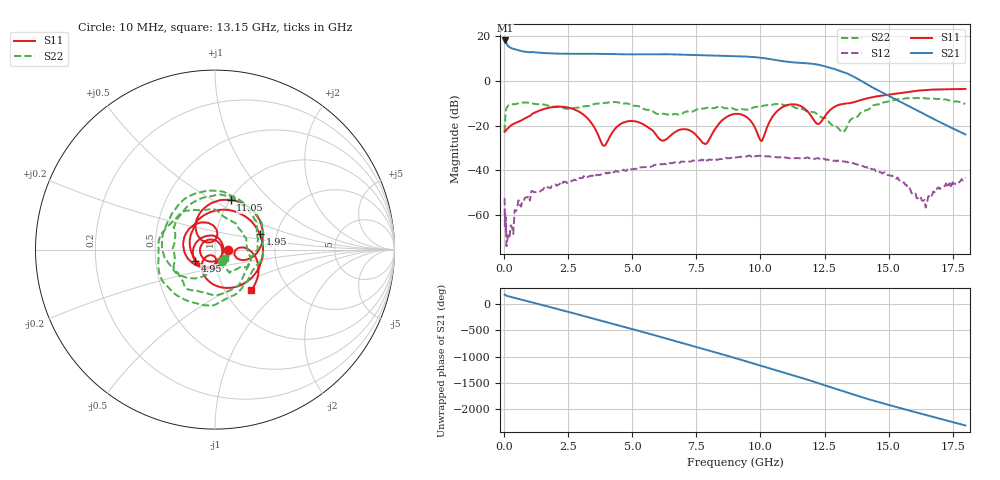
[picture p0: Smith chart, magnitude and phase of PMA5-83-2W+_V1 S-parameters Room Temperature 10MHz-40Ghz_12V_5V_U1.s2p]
!Mini-Circuits Laboratory
!S-Parameters
!Model: US-AMP-1
!Run / Lot / Date Code: N/A /  / N/A
!Fixture: ON TB-
!Network Analyzer: NFA N8975A;  Serial number: 74408
!Date: 12/1/2023 at 8:03:08 AM
!No.: Unit# 1 (#1)
!Tested with:
!Condition 2: Vdd = +12V; Vg2= +5V; Idd= 400mA
# Hz  S  dB  R  50
!Frequency  S11 dB  S11 Deg  S21 dB  S21 Deg  S12 dB  S12 Deg  S22 dB  S22 Deg
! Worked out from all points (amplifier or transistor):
!   368 points, 10 MHz to 18 GHz, reference 50 ohm
!   highest |S21| = 18.2 dB at 20 MHz (marker M1)
!   |S21| within 3 dB of that: start of sweep to 198.7 MHz
!   unconditionally stable (mu >= 1): start of sweep to end of sweep
!   at 2.7 GHz: K = 18.17, MAG = 12.7 dB, |S12| = -44.5 dB
!   at 8.85 GHz: K = 6.53, MAG = 11.6 dB, |S12| = -34.3 dB
!   at 18 GHz: K = 559.16, MAG = -20.9 dB, |S12| = -43.1 dB
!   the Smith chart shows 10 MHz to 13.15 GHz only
!   S11 on the Smith chart (normalised r, x): 10 MHz: 1.16, -0.00; 1.95 GHz: 1.63, +0.30; 4.95 GHz: 0.79, -0.10; 11.05 GHz: 1.01, +0.61; 13.15 GHz: 1.31, -0.66
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1e7  -22.68 -0.5  17.95 177.8  -52.38 -62.5  -22.73 -57.9
2e7  -22.62 -3.8  18.17 174.4  -65.67 23.9  -19.73 -85.4
4.5e8  -18.71 -130.9  14.12 108.2  -58.23 52.9  -10.29 145.9
1.1e9  -14.57 124.1  13.01 27.2  -49.12 -39.4  -10.05 72.8
1.95e9  -11.56 18.7  12.33 -81.3  -46.48 -144.7  -11.47 -1.4
2.55e9  -12.01 -47.0  12.22 -158.0  -45.09 138.9  -12.26 -36.4
3.05e9  -14.69 -98.4  12.22 137.2  -43.40 76.6  -11.40 -60.0
4.05e9  -26.41 -85.3  12.09 5.7  -40.94 -45.2  -9.56 -130.2
4.95e9  -17.86 -151.1  11.95 -112.5  -39.45 -157.2  -10.56 154.9
5.5e9  -19.85 142.9  12.01 174.6  -38.47 130.5  -12.70 106.2
6.05e9  -25.89 33.6  12.04 100.4  -37.19 62.9  -14.71 60.9
6.75e9  -22.21 -127.0  11.91 4.7  -36.63 -29.8  -14.91 14.5
7.4e9  -23.22 130.4  11.65 -84.3  -35.61 -113.8  -13.31 -42.0
8.15e9  -22.98 -77.0  11.41 172.8  -35.15 147.1  -12.15 -105.6
9.05e9  -14.65 153.0  11.12 46.5  -34.17 26.0  -12.84 -168.3
9.95e9  -25.40 89.7  10.53 -84.3  -33.36 -97.5  -11.33 140.1
1.05e10  -15.45 130.1  9.59 -164.8  -33.85 -175.4  -10.51 93.4
1.105e10  -10.71 72.5  8.64 117.0  -34.22 110.5  -10.90 46.2
1.205e10  -16.90 -22.1  7.70 -31.4  -34.50 -31.9  -13.83 -27.7
1.315e10  -10.38 -48.7  4.39 154.5  -35.66 152.8  -22.61 -41.1
1.505e10  -6.00 125.0  -6.81 -122.7  -42.20 -104.5  -9.00 -118.3
1.8e10  -3.51 178.2  -23.85 -146.8  -43.12 84.4  -10.18 58.0
